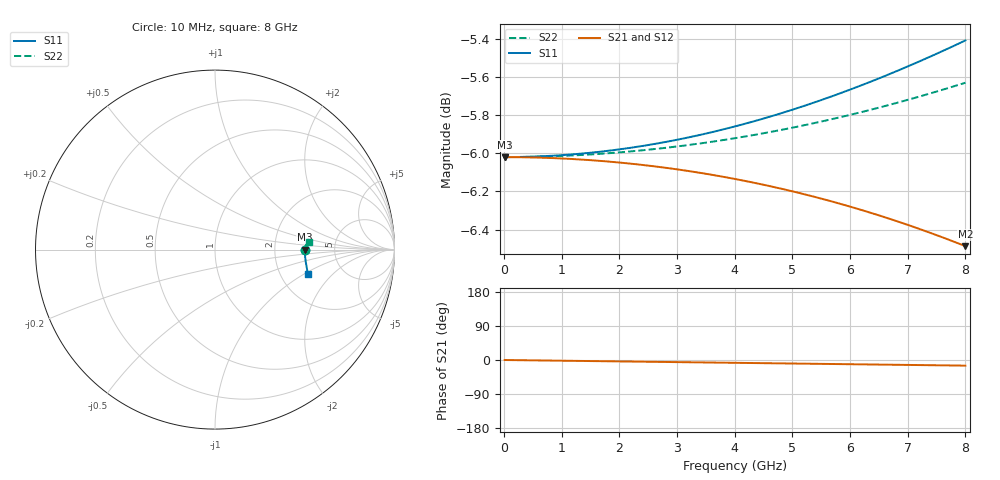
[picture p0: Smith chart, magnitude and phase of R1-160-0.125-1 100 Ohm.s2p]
!version-2
!date-03.2021
# MHz S RI R 50
!Freq ReS11 ImS11 ReS21 ImS21 ReS12 ImS12 ReS22 ImS22
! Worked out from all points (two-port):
!   800 points, 10 MHz to 8 GHz, reference 50 ohm
!   highest |S21| = -6.02 dB at 10 MHz (marker M1); lowest = -6.5 dB at 8 GHz (marker M2)
!   |S21| within 3 dB of the highest: start of sweep to end of sweep
!   lowest |S11| = -6.0 dB at 10 MHz (marker M3), VSWR 3.00, Z = 150 - j0.063 ohm
!   |S11| at or under -10 dB: nowhere
!   |S22| runs from -6.0 to -5.6 dB; largest |S21 - S12| = 0
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10  0.5 -0.000157  0.5 -0.000164  0.5 -0.000164  0.5 5.65e-05
50  0.5 -0.000787  0.5 -0.000818  0.5 -0.000818  0.5 0.000282
680  0.5002 -0.0107  0.4997 -0.0111  0.4997 -0.0111  0.5002 0.00384
1010  0.5003 -0.0159  0.4993 -0.0165  0.4993 -0.0165  0.5003 0.0057
1350  0.5006 -0.0213  0.4988 -0.0221  0.4988 -0.0221  0.5006 0.00761
1680  0.5009 -0.0266  0.4981 -0.0274  0.4981 -0.0274  0.5009 0.00946
2010  0.5014 -0.0318  0.4973 -0.0327  0.4973 -0.0327  0.5013 0.0113
2340  0.5018 -0.0372  0.4963 -0.0381  0.4963 -0.0381  0.5018 0.0132
2680  0.5024 -0.0427  0.4952 -0.0435  0.4952 -0.0435  0.5023 0.015
3010  0.503 -0.0481  0.4939 -0.0488  0.4939 -0.0488  0.503 0.0169
3340  0.5037 -0.0535  0.4925 -0.054  0.4925 -0.054  0.5036 0.0187
3670  0.5044 -0.059  0.491 -0.0592  0.491 -0.0592  0.5044 0.0205
4010  0.5052 -0.0648  0.4892 -0.0644  0.4892 -0.0644  0.5053 0.0224
4670  0.507 -0.0761  0.4854 -0.0745  0.4854 -0.0745  0.5071 0.0259
5000  0.5079 -0.0819  0.4833 -0.0795  0.4833 -0.0795  0.5082 0.0277
5340  0.509 -0.0879  0.481 -0.0846  0.481 -0.0846  0.5094 0.0295
6000  0.5111 -0.0999  0.4761 -0.0942  0.4761 -0.0942  0.5118 0.0329
6670  0.5134 -0.1124  0.4706 -0.1037  0.4706 -0.1037  0.5147 0.0364
7070  0.5148 -0.1201  0.467 -0.1092  0.467 -0.1092  0.5165 0.0383
7470  0.5163 -0.1279  0.4633 -0.1145  0.4633 -0.1145  0.5184 0.0403
7960  0.5181 -0.1377  0.4584 -0.1209  0.4584 -0.1209  0.521 0.0427
8000  0.5182 -0.1385  0.458 -0.1214  0.458 -0.1214  0.5212 0.0428
